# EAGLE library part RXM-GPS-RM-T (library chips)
The RM Series GPS receiver module is a self-contained high-performance Global Positioning System receiver
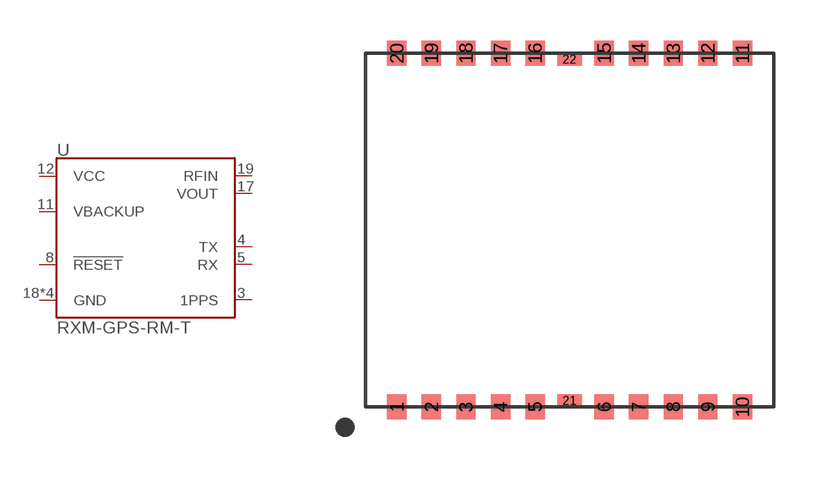
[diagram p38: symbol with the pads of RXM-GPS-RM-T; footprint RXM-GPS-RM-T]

Designator prefix U

## RXM-GPS-RM-T (DIGIKEY: RXM-GPS-RM-TCT-ND)  [RXM-GPS-RM-T]
3  1PPS
4  TX
5  RX
8  !RESET
11  VBACKUP
12  VCC
17  VOUT
18  GND
19  RFIN
20  GND
21  GND
22  GND

## Footprint RXM-GPS-RM-T (pad centres in mm)
smd 0.711 x 0.914: 1 -6.35,-6.502; 2 -5.08,-6.502; 3 -3.81,-6.502; 4 -2.54,-6.502; 5 -1.27,-6.502; 6 1.27,-6.502; 7 2.54,-6.502; 8 3.81,-6.502; 9 5.08,-6.502; 10 6.35,-6.502; 11 6.35,6.502; 12 5.08,6.502; 13 3.81,6.502; 14 2.54,6.502; 15 1.27,6.502; 16 -1.27,6.502; 17 -2.54,6.502; 18 -3.81,6.502; 19 -5.08,6.502; 20 -6.35,6.502
smd 0.914 x 0.457: 21 0,-6.274; 22 0,6.274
